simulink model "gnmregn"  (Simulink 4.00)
settings: Solver=ode45  StartTime=0.0  StopTime=Tstop  MaxStep=step_max  RelTol=1e-3
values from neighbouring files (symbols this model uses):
  CE = 2*pi*CM    (= 240.017678734)    [gnm_i.m]
  CM = 38.2    [gnm_i.m]
  int_regi = 0    [gnmregi_i.m]
  int_regn = 0    [gnmregn_i.m]    (also in lsg_gnmregnss_ini.m)
  J = 0.012    [gnm_i.m]
  MW = 10    [gnmbeobreg_i.m]    (also in gnmbeob_i.m; gnmregn_i.m = 100; gnm_i.m = 0; lsg_gnmregnss_ini.m = 100)
  PsiN = 0.04    [gnm_i.m]
  RA = 0.250    (= 0.25)    [gnm_i.m]
  T_MW = 0.4    [gnmbeobreg_i.m]    (also in gnmbeob_i.m; gnmregn_i.m = 0.1; gnm_i.m = 0; lsg_gnmregnss_ini.m = 0.1)
  T_Ri = TA    [gnmregi_i.m]
  T_Rn = 4*2*T_t    [gnmregn_i.m]    (also in lsg_gnmregnss_ini.m = 4^2*2*T_t)
  T_t = 0.0001    [gnmbeobreg_i.m]    (also in gnmbeob_i.m; gnmregi_i.m)
  TA = LA / RA    (= 0.016)    [gnm_i.m]
  V_Ri = LA / (2*T_t)    [gnmregi_i.m]
  V_Rn = 2*pi*J / (CM*PsiN*2*2*T_t)    [gnmregn_i.m]    (also in lsg_gnmregnss_ini.m = 2*pi*J / (CM*PsiN*4*2*T_t))
libraries: simulink3 x1

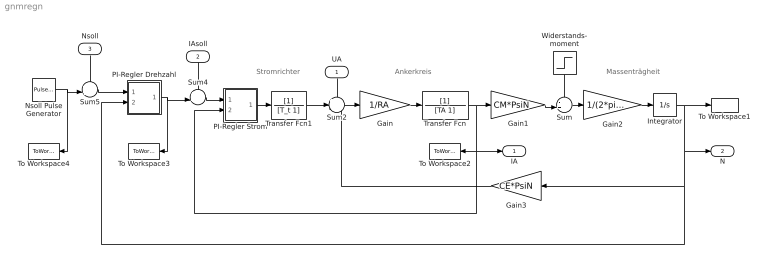
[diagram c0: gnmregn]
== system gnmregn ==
  note: Massenträgheit
  note: Ankerkreis
  note: Stromrichter
  UA : Inport  Orientation=down  Port=1
  IAsoll : Inport  Orientation=down  Port=2  PortDimensions=1
  Nsoll : Inport  Orientation=down  Port=3  PortDimensions=1
  Gain : Gain  Gain=1/RA  Multiplication=Element-wise(K.*u)  SaturateOnIntegerOverflow=on
  Gain1 : Gain  Gain=CM*PsiN  Multiplication=Element-wise(K.*u)  SaturateOnIntegerOverflow=on
  Gain2 : Gain  Gain=1/(2*pi*J)  Multiplication=Element-wise(K.*u)  SaturateOnIntegerOverflow=on
  Gain3 : Gain  Orientation=left  Gain=CE*PsiN  Multiplication=Element-wise(K.*u)  SaturateOnIntegerOverflow=on
  Integrator : Integrator  ExternalReset=none  InitialConditionSource=internal  InitialCondition=0  LimitOutput=off  UpperSaturationLimit=inf  LowerSaturationLimit=-inf  ShowSaturationPort=off  ShowStatePort=off  AbsoluteTolerance=auto
  Nsoll Pulse Generator : simulink3/Sources/Pulse Generator  period=T_Nsoll  duty=50  amplitude=N_soll  start=0
  PI-Regler Drehzahl : Subsystem  mask(PI-Regler){V_R=V_Rn, T_n=T_Rn, int_R=int_regn}
      mask prompts: V_R "Verstärkungsfaktor V_R"; T_n "Nachstellzeit T_n"; int_R "Startwert Regler-Integrator"
      mask help: 1 + s*T_n 1 + s*T_n Übertragungsfunktion: G_R = V_R * ------------------ = K_R * ------------------ s*T_n s
  PI-Regler Strom : Subsystem  mask(PI-Regler){V_R=V_Ri, T_n=T_Ri, int_R=int_regi}
      mask prompts: V_R "Verstärkungsfaktor V_R"; T_n "Nachstellzeit T_n"; int_R "Startwert Regler-Integrator"
      mask help: 1 + s*T_n 1 + s*T_n Übertragungsfunktion: G_R = V_R * ------------------ = K_R * ------------------ s*T_n s
  Sum : Sum  Inputs=-+|  SaturateOnIntegerOverflow=on
  Sum2 : Sum  Inputs=++-  SaturateOnIntegerOverflow=on
  Sum4 : Sum  Inputs=++|  SaturateOnIntegerOverflow=on
  Sum5 : Sum  Inputs=++|  SaturateOnIntegerOverflow=on
  To Workspace1 : ToWorkspace  VariableName=N  SampleTime=-1  SaveFormat=Array
  To Workspace2 : ToWorkspace  VariableName=IA  SampleTime=-1  SaveFormat=Array
  To Workspace3 : ToWorkspace  VariableName=IAsoll  SampleTime=-1  SaveFormat=Array
  To Workspace4 : ToWorkspace  VariableName=Nsoll  SampleTime=-1  SaveFormat=Array
  Transfer Fcn : TransferFcn  Numerator=[1]  Denominator=[TA 1]  Realization=auto  AbsoluteTolerance=auto
  Transfer Fcn1 : TransferFcn  Numerator=[1]  Denominator=[T_t 1]  Realization=auto  AbsoluteTolerance=auto
  Widerstands- moment : Step  Orientation=down  Time=T_MW  Before=0  After=MW  SampleTime=0
  IA : Outport  Port=1
  N : Outport  Port=2
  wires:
  PI-Regler Strom/1(Reglerausgang) -> Transfer Fcn1/1
  Gain/1 -> Transfer Fcn/1
  Sum2/1 -> Gain/1
  Gain1/1 -> Sum/2
  Widerstands- moment/1 -> Sum/1
  Sum/1 -> Gain2/1
  Gain2/1 -> Integrator/1
  Integrator/1 -> To Workspace1/1, N/1, Gain3/1, PI-Regler Drehzahl/2(Istwert)
  UA/1 -> Sum2/1
  Gain3/1 -> Sum2/3
  Transfer Fcn/1 -> Gain1/1, To Workspace2/1, IA/1, PI-Regler Strom/2(Istwert)
  Transfer Fcn1/1 -> Sum2/2
  IAsoll/1 -> Sum4/1
  Sum4/1 -> PI-Regler Strom/1(Sollwert)
  PI-Regler Drehzahl/1(Reglerausgang) -> Sum4/2, To Workspace3/1
  Nsoll/1 -> Sum5/1
  Sum5/1 -> PI-Regler Drehzahl/1(Sollwert)
  Nsoll Pulse Generator/1 -> To Workspace4/1, Sum5/2

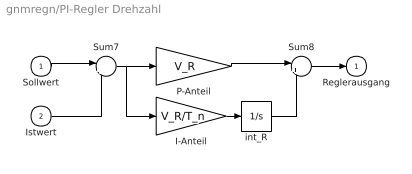
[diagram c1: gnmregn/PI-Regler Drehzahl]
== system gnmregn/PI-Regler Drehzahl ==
  Sollwert : Inport  Port=1
  Istwert : Inport  Port=2
  I-Anteil : Gain  Gain=V_R/T_n  Multiplication=Element-wise(K.*u)  SaturateOnIntegerOverflow=on
  P-Anteil : Gain  Gain=V_R  Multiplication=Element-wise(K.*u)  SaturateOnIntegerOverflow=on
  Sum7 : Sum  Inputs=|+-  SaturateOnIntegerOverflow=on
  Sum8 : Sum  Inputs=|++  SaturateOnIntegerOverflow=on
  int_R : Integrator  ExternalReset=none  InitialConditionSource=internal  InitialCondition=int_R  LimitOutput=off  UpperSaturationLimit=inf  LowerSaturationLimit=-inf  ShowSaturationPort=off  ShowStatePort=off  AbsoluteTolerance=auto
  Reglerausgang : Outport  Port=1  InitialOutput=0
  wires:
  P-Anteil/1 -> Sum8/1
  I-Anteil/1 -> int_R/1
  int_R/1 -> Sum8/2
  Sum8/1 -> Reglerausgang/1
  Sum7/1 -> P-Anteil/1, I-Anteil/1
  Istwert/1 -> Sum7/2
  Sollwert/1 -> Sum7/1

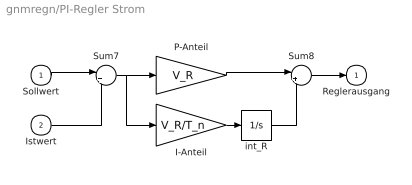
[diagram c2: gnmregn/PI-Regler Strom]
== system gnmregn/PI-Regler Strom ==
  Sollwert : Inport  Port=1
  Istwert : Inport  Port=2
  I-Anteil : Gain  Gain=V_R/T_n  Multiplication=Element-wise(K.*u)  SaturateOnIntegerOverflow=on
  P-Anteil : Gain  Gain=V_R  Multiplication=Element-wise(K.*u)  SaturateOnIntegerOverflow=on
  Sum7 : Sum  Inputs=|+-  SaturateOnIntegerOverflow=on
  Sum8 : Sum  Inputs=|++  SaturateOnIntegerOverflow=on
  int_R : Integrator  ExternalReset=none  InitialConditionSource=internal  InitialCondition=int_R  LimitOutput=off  UpperSaturationLimit=inf  LowerSaturationLimit=-inf  ShowSaturationPort=off  ShowStatePort=off  AbsoluteTolerance=auto
  Reglerausgang : Outport  Port=1  InitialOutput=0
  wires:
  P-Anteil/1 -> Sum8/1
  I-Anteil/1 -> int_R/1
  int_R/1 -> Sum8/2
  Sum8/1 -> Reglerausgang/1
  Sum7/1 -> P-Anteil/1, I-Anteil/1
  Istwert/1 -> Sum7/2
  Sollwert/1 -> Sum7/1
